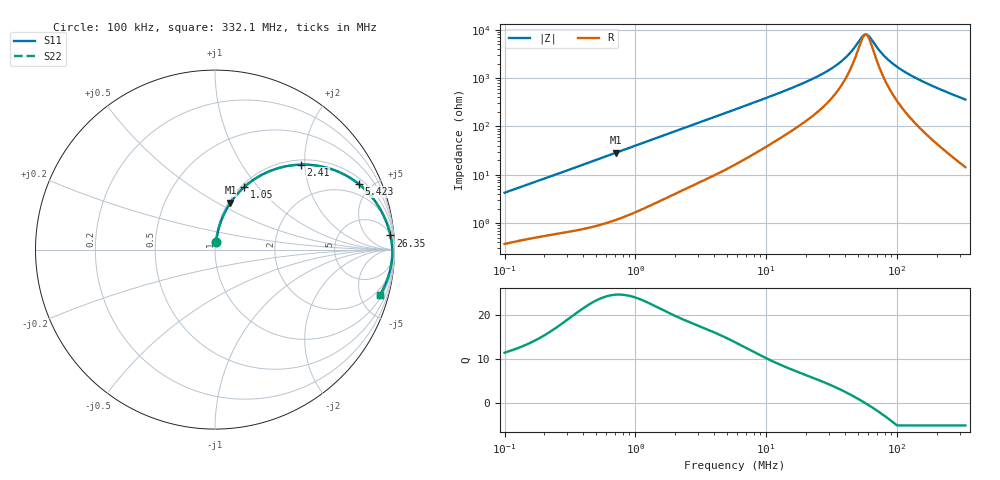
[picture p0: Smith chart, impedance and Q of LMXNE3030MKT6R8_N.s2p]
! LMXNE3030MKT6R8_N  S-PARAMETER MODEL  ( General Type )
! Model Generated by TAIYO YUDEN Corporation (http://www.ty-top.com)
! Version 1.0
! TAIYO YUDEN Control No. 191023NI43SB-FBB
! Copyright(c) 2019 TAIYO YUDEN CO.,LTD. All Rights Reserved.
! Product Description (link to TY-COMPAS)
! https://ds.yuden.co.jp/TYCOMPAS/or/detail?pn=LMXNE3030MKT6R8MN&u=M
! Products Name : Inductors
! Characteristics :
!  Inductance : 6.8 uH , SRF(min) : 43 MHz , DC Resistance(max) : 0.228 Ohm
!  Rated Current : Saturation :850 mA , Temp Rise : 890 mA
!  Case Size : 3.0 x 3.0 / 0.118 x 0.118 [mm/inch] , Thickness : 1.2 / 0.047 [mm/inch]
!  (Conditions: Temperature = 25 degC , DC Bias Current/Voltage = 0A / 0V)
! External Node Assignments :
!  1  o---GGG---o  2
! GND o---------o GND
! Frequency Range : 0.1MHz  -  332.076389MHz  [ 402 STEP ]
# MHz S RI R 50
! Freq[MHz].  S11 Real  S11 Imag  S21 Real  S21 Imag  S12 Real  S12 Imag  S22 Real  S22 Imag
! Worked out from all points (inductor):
!   401 points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, 100 kHz to 332.1 MHz, reference 50 ohm
!   read as one part in series: L = 6.7 uH near 104.1 kHz
!   highest Q = 24.5 at 714.3 kHz (marker M1), where L = 6.44 uH
!   self-resonance near 56.93 MHz
!   S11 on the Smith chart (normalised r, x): 100 kHz: 1.01, +0.09; 1.05 MHz: 1.04, +0.84; 2.41 MHz: 1.10, +1.90; 5.423 MHz: 1.30, +4.21; 26.35 MHz: 6, +23; 332.1 MHz: 1.29, -7.20
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0.1  0.0055 0.0421  0.9945 -0.0421  0.9945 -0.0421  0.0055 0.0421
0.388873  0.0314 0.1524  0.9686 -0.1524  0.9686 -0.1524  0.0314 0.1524
0.714332  0.0862 0.2609  0.9138 -0.2609  0.9138 -0.2609  0.0862 0.2609
1.049927  0.1619 0.3478  0.8381 -0.3478  0.8381 -0.3478  0.1619 0.3478
1.512219  0.2769 0.4248  0.7231 -0.4248  0.7231 -0.4248  0.2769 0.4248
2.410382  0.4773 0.4735  0.5227 -0.4735  0.5227 -0.4735  0.4773 0.4735
3.471695  0.6416 0.4507  0.3584 -0.4507  0.3584 -0.4507  0.6416 0.4507
5.422627  0.8006 0.3659  0.1994 -0.3659  0.1994 -0.3659  0.8006 0.3659
5.762607  0.8172 0.3519  0.1828 -0.3519  0.1828 -0.3519  0.8172 0.3519
10.16496  0.9206 0.2252  0.0794 -0.2252  0.0794 -0.2252  0.9206 0.2252
22.4092  0.9727 0.0984  0.0273 -0.0984  0.0273 -0.0984  0.9727 0.0984
26.35428  0.9775 0.079  0.0225 -0.079  0.0225 -0.079  0.9775 0.079
38.73557  0.9847 0.038  0.0153 -0.038  0.0153 -0.038  0.9847 0.038
44.64076  0.9862 0.024  0.0138 -0.024  0.0138 -0.024  0.9862 0.024
53.57466  0.9874 0.00656  0.0126 -0.00656  0.0126 -0.00656  0.9874 0.00656
56.93361  0.9877 0.000759  0.0123 -0.000759  0.0123 -0.000759  0.9877 0.000759
61.74206  0.9878 -0.007  0.0122 0.007  0.0122 0.007  0.9878 -0.007
74.09842  0.9876 -0.0248  0.0124 0.0248  0.0124 0.0248  0.9876 -0.0248
87.14324  0.9868 -0.0413  0.0132 0.0413  0.0132 0.0413  0.9868 -0.0413
108.91  0.9844 -0.0657  0.0156 0.0657  0.0156 0.0657  0.9844 -0.0657
144.6476  0.9785 -0.1013  0.0215 0.1013  0.0215 0.1013  0.9785 -0.1013
332.0764  0.9199 -0.2522  0.0801 0.2522  0.0801 0.2522  0.9199 -0.2522
